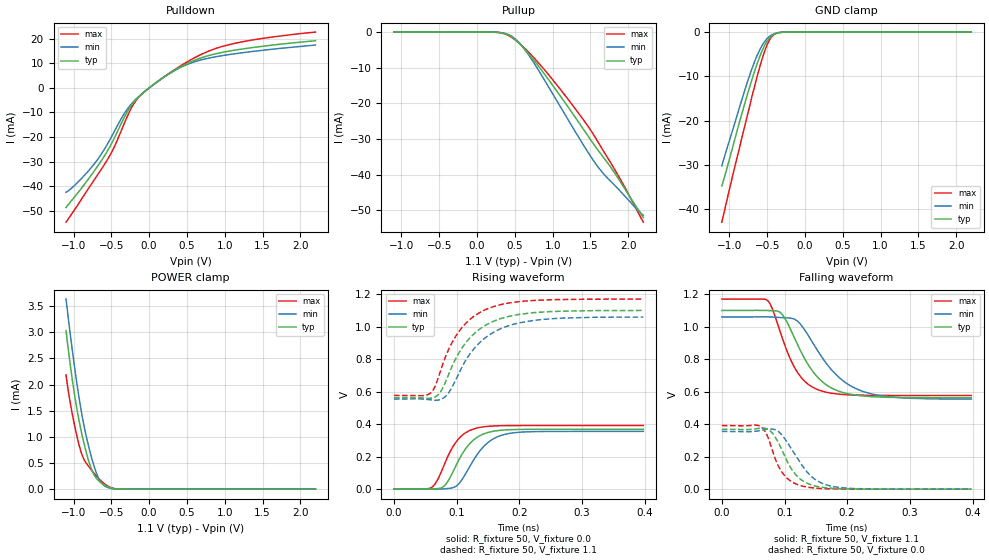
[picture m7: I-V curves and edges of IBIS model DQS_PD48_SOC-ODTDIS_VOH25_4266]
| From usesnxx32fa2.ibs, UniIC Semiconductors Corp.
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| DQS_PD48_SOC-ODTDIS_VOH25_4266
| (48 Ohm Pulldown, SOC ODT disabled setting, VOH=VDDQ/2.5 cal. point, 3200-4266Mbps)
[Model]   DQS_PD48_SOC-ODTDIS_VOH25_4266
Model_type   I/O
Vinl = 160.000mV
Vinh = 280.000mV
Vmeas = 220.000mV
Vref = 0.0mV
Cref = 0.0pF
|   typ   min   max
|C_comp   0.849pF   0.799pF   0.899pF
C_comp_pullup   0.4245pF   0.3995pF   0.4495pF
C_comp_pulldown   0.4245pF   0.3995pF   0.4495pF
| Note: C_comp changes when the ODT circuit is enabled.
[Model Spec]
| Input threshold voltage corners
Vinl   0.1600V   0.1520V   0.1740V
Vinh   0.2800V   0.2720V   0.2940V
| Measurement voltage corners
Vmeas   0.2200V   0.2120V   0.2340V
| Timing spec test load voltage corners
Vref   0.0000V   0.0000V   0.0000V
| Dynamic Overshoot Parameters from LPDDR4 Specification
D_overshoot_ampl_h   0.30   NA   NA
D_overshoot_ampl_l   0.30   NA   NA
D_overshoot_area_h   0.1n   NA   NA
D_overshoot_area_l   0.1n   NA   NA
[Voltage Range]   1.1000V   1.0600V   1.1700V
[Pullup Reference]   1.1000V   1.0600V   1.1700V
| Junction Temperature (Ambient temp is 35C typ 95C min -40C max)
[Temperature Range]   50.0   110.0   -40.0
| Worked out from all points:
|   slope of the pulldown table from 0 to 0.165 V, typ, clamps not added: 43.8 ohm
|   slope of the pullup table from 0 to 0.165 V, typ, clamps not added: 17.7 kohm
|   GND clamp passes 1 mA (typ) near -0.45 V on its own axis
|   POWER clamp passes 1 mA (typ) near -0.88 V on its own axis
|   rising waveform, R_fixture 50, V_fixture 0.0: 20-80 % time 34.8ps typ, 38.4ps min, 31.7ps max; typ from 0.001 V to 0.368 V
|   falling waveform, R_fixture 50, V_fixture 1.1: 20-80 % time 49.2ps typ, 61.8ps min, 39ps max; typ from 1.1 V to 0.563 V
|   rising waveform, R_fixture 50, V_fixture 1.1: 20-80 % time 56.1ps typ, 59.2ps min, 51.8ps max; typ from 0.563 V to 1.1 V
|   falling waveform, R_fixture 50, V_fixture 0.0: 20-80 % time 32.7ps typ, 40ps min, 27.1ps max; typ from 0.368 V to 0.001 V
[Pulldown]
|   Voltage   I(typ)   I(min)   I(max)
-1.1V     -48.66mA   -42.43mA   -54.64mA
-783.2mV  -36.22mA   -33.06mA   -40.03mA
-638mV    -29.88mA   -27.18mA   -33.36mA
-525.8mV  -24.27mA   -21.44mA   -27.81mA
-331.1mV  -12.13mA   -10.56mA   -14.58mA
-202.4mV  -5.787mA   -5.454mA   -6.434mA
-110mV    -2.844mA   -2.792mA   -2.874mA
48.4mV    1.124mA    1.121mA    1.122mA
467.5mV   9.38mA     9.054mA    9.949mA
883.3mV   13.89mA    12.68mA    16.05mA
1.408V    16.57mA    14.97mA    19.69mA
2.2V      19.18mA    17.44mA    22.7mA
[GND Clamp]
|   Voltage   I(typ)   I(min)   I(max)
-1.1V     -34.75mA   -30.22mA   -42.92mA
-941.6mV  -25.02mA   -21.25mA   -31.33mA
-799.7mV  -16.31mA   -13.32mA   -21.43mA
-723.8mV  -11.94mA   -9.346mA   -16.11mA
-664.4mV  -8.74mA    -6.576mA   -12.08mA
-591.8mV  -5.257mA   -3.788mA   -7.499mA
-519.2mV  -2.565mA   -1.834mA   -3.663mA
-469.7mV  -1.359mA   -985.3uA   -1.791mA
-413.6mV  -565.5uA   -416.3uA   -623.4uA
-347.6mV  -154.9uA   -117.2uA   -136.4uA
-242mV    -10.09uA   -9.282uA   -5.68uA
2.2V      0A         0A         0A
[Pullup]
|   Voltage   I(typ)   I(min)   I(max)
-1.1V     4.106uA    7.431uA    1.361uA
266.2mV   -68.96uA   -66.66uA   -71.79uA
385mV     -549.2uA   -456.7uA   -657.5uA
503.8mV   -2.098mA   -1.888mA   -2.196mA
606.1mV   -4.22mA    -4.209mA   -4.061mA
738.1mV   -7.54mA    -8.193mA   -6.899mA
1.088V    -17.54mA   -20.45mA   -15.71mA
1.458V    -28.85mA   -33.42mA   -26.13mA
1.589V    -32.85mA   -37.56mA   -30.49mA
1.675V    -35.26mA   -39.82mA   -33.5mA
1.956V    -44.08mA   -46.07mA   -43.63mA
2.2V      -52.05mA   -51.41mA   -53.39mA
[POWER Clamp]
|   Voltage   I(typ)   I(min)   I(max)
-1.1V     3.033mA    3.633mA    2.184mA
-1.041V   2.345mA    2.929mA    1.625mA
-981.2mV  1.753mA    2.275mA    1.183mA
-911.9mV  1.2mA      1.61mA     764.4uA
-852.5mV  818.2uA    1.148mA    543.6uA
-776.6mV  434.1uA    683.3uA    390.2uA
-710.6mV  232.2uA    359uA      273.1uA
-654.5mV  142.7uA    170.4uA    185.9uA
-598.4mV  83.64uA    71.96uA    113uA
-482.9mV  15.71uA    9.515uA    19.53uA
-364.1mV  1.102uA    823.2nA    868.3nA
2.2V      0A         0A         0A
[Ramp]
|   typ   min   max
| 20% - 80%
dV/dt_r   220.63m/34.77p   212.96m/38.41p   234.70m/31.71p
dV/dt_f   322.27m/49.23p   303.39m/61.76p   356.00m/38.99p
| 25% - 75%
|dV/dt_r   183.86m/27.68p   177.47m/30.60p   195.58m/25.19p
|dV/dt_f   268.56m/39.26p   252.82m/49.26p   296.66m/31.04p
R_load = 50
[Rising Waveform]
R_fixture = 50
V_fixture = 0.0
|   Time   V(typ)   V(min)   V(max)
0s        642.1uV    518.8uV    473.3uV
59ps      752.9uV    89.61uV    7.998mV
68ps      2.748mV    -236.7uV   46.15mV
78ps      12.91mV    1.096mV    129.3mV
103ps     175.6mV    30.58mV    308.5mV
117ps     262.1mV    111.9mV    353mV
132ps     316.9mV    208.7mV    375.6mV
156ps     354.2mV    303.5mV    388.2mV
187ps     366.2mV    344.6mV    391.3mV
398ps     368.4mV    355.5mV    391.6mV
[Falling Waveform]
R_fixture   = 50
V_fixture   = 1.1
V_fixture_min = 1.06
V_fixture_max = 1.17
|   Time   V(typ)   V(min)   V(max)
0s        1.1V       1.06V      1.17V
73ps      1.1V       1.061V     1.161V
81ps      1.099V     1.059V     1.106V
96ps      1.077V     1.056V     935.8mV
117ps     921mV      1.044V     742.1mV
132ps     804.2mV    981.7mV    665.2mV
153ps     688.7mV    851.4mV    612.8mV
187ps     602.7mV    688mV      585.1mV
228ps     572.8mV    598.1mV    578.1mV
398ps     562.9mV    554.3mV    576.7mV
[Rising Waveform]
R_fixture   = 50
V_fixture   = 1.1
V_fixture_min = 1.06
V_fixture_max = 1.17
|   Time   V(typ)   V(min)   V(max)
0s        562.8mV    553.9mV    576.6mV
57ps      559mV      549.9mV    587.4mV
66ps      568.1mV    547mV      635.7mV
79ps      631.2mV    560.3mV    781.3mV
94ps      766.8mV    636.3mV    910.9mV
112ps     887.5mV    775.9mV    1.009V
131ps     967.2mV    878.9mV    1.073V
153ps     1.023V     951.5mV    1.116V
228ps     1.088V     1.041V     1.162V
398ps     1.1V       1.059V     1.17V
[Falling Waveform]
R_fixture = 50
V_fixture = 0.0
|   Time   V(typ)   V(min)   V(max)
0s        368.5mV    355.6mV    391.7mV
58ps      374.1mV    358.9mV    392.2mV
75ps      365.5mV    370.5mV    305.8mV
87ps      309.2mV    362.8mV    169.8mV
97ps      232.5mV    328.3mV    99.23mV
112ps     119.2mV    242.5mV    45.03mV
128ps     55.03mV    147mV      19.78mV
151ps     18.4mV     54.75mV    6.377mV
182ps     4.771mV    13.9mV     1.712mV
398ps     686.6uV    587.3uV    490.8uV
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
